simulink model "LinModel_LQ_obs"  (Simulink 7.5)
settings: Solver=ode45  StartTime=0.0  StopTime=10.0  RelTol=1e-3
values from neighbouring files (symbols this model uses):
  dX0 = [0 0 0.55 0]'    [Exercises05.m]
  K = lqr(A,B,C'*Q*C,R)    [Exercises05.m]
  Lobs = - place(A',C',[-20 -20 -25 -25])'    [Exercises05.m]
undefined symbols (not defined in the file or in its folder): A, B, C

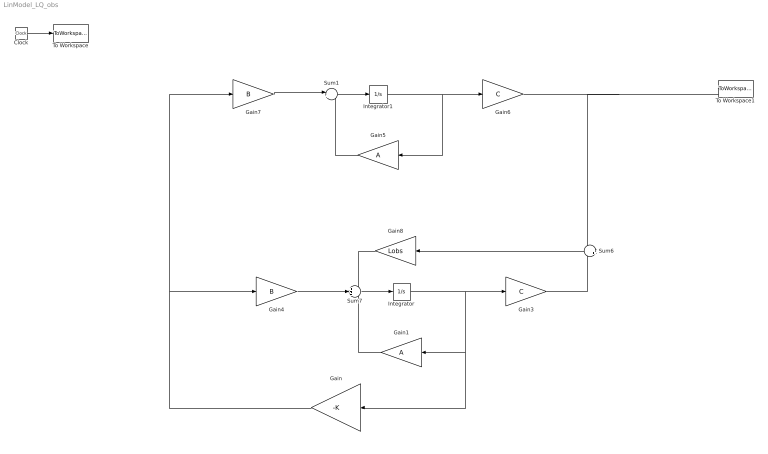
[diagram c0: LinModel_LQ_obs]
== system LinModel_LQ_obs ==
  Clock : Clock
  Gain : Gain  Gain=-K  Multiplication=Matrix(K*u)  ParameterDataType=fixdt(1, 16)  ParameterScaling=2^0  OutDataType=fixdt(1, 16)  OutScaling=2^0
  Gain1 : Gain  Gain=A  Multiplication=Matrix(K*u)  ParameterDataType=sfix(16)  ParameterScaling=2^0  OutDataType=sfix(16)  OutScaling=2^0
  Gain3 : Gain  Gain=C  Multiplication=Matrix(K*u)  ParameterDataType=sfix(16)  ParameterScaling=2^0  OutDataType=sfix(16)  OutScaling=2^0
  Gain4 : Gain  Gain=B  Multiplication=Matrix(K*u)  ParameterDataType=sfix(16)  ParameterScaling=2^0  OutDataType=sfix(16)  OutScaling=2^0
  Gain5 : Gain  Gain=A  Multiplication=Matrix(K*u)  ParameterDataType=sfix(16)  ParameterScaling=2^0  OutDataType=sfix(16)  OutScaling=2^0
  Gain6 : Gain  Gain=C  Multiplication=Matrix(K*u)  ParameterDataType=sfix(16)  ParameterScaling=2^0  OutDataType=sfix(16)  OutScaling=2^0
  Gain7 : Gain  Gain=B  Multiplication=Matrix(K*u)  ParameterDataType=sfix(16)  ParameterScaling=2^0  OutDataType=sfix(16)  OutScaling=2^0
  Gain8 : Gain  Gain=Lobs  Multiplication=Matrix(K*u)  ParameterDataType=sfix(16)  ParameterScaling=2^0  OutDataType=sfix(16)  OutScaling=2^0
  Integrator : Integrator  InitialCondition=[0 0 0 0]'
  Integrator1 : Integrator  InitialCondition=dX0
  Sum1 : Sum  Inputs=|++  OutDataType=sfix(16)  OutScaling=2^0
  Sum6 : Sum  Inputs=-+  OutDataType=sfix(16)  OutScaling=2^0
  Sum7 : Sum  Inputs=+++  OutDataType=sfix(16)  OutScaling=2^0
  To Workspace : ToWorkspace  VariableName=time  SampleTime=-1  SaveFormat=Array
  To Workspace1 : ToWorkspace  VariableName=dy  SampleTime=-1  SaveFormat=Array
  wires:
  Clock/1 -> To Workspace/1
  Gain/1 -> Gain4/1, Gain7/1
  Integrator/1 -> Gain3/1, Gain1/1, Gain/1
  Sum7/1 -> Integrator/1
  Gain3/1 -> Sum6/2
  Sum6/1 -> Gain8/1
  Gain8/1 -> Sum7/1
  Gain1/1 -> Sum7/3
  Gain4/1 -> Sum7/2
  Integrator1/1 -> Gain6/1, Gain5/1
  Sum1/1 -> Integrator1/1
  Gain5/1 -> Sum1/2
  Gain7/1 -> Sum1/1
  Gain6/1 -> To Workspace1/1, Sum6/1
